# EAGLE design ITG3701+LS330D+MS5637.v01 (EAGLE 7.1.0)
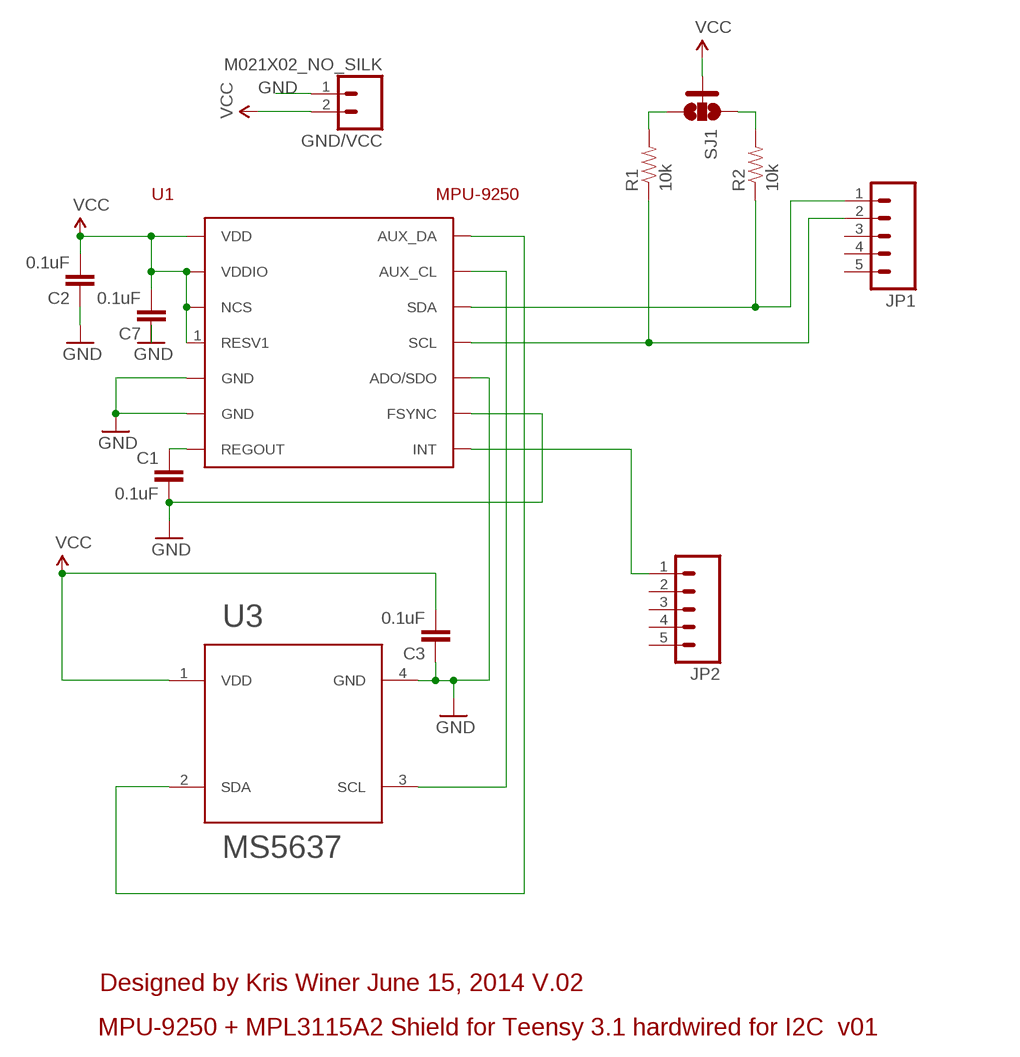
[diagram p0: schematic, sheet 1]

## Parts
C1  0.1uF  4.7UF-6.3V-10%(0603)0603  [0603-CAP]
C2  0.1uF  0.22UF-25V-10%(0603)  [0603-CAP]
C3  0.1uF  0.22UF-25V-10%(0603)  [0603-CAP]
C7  0.1uF  0.22UF-25V-10%(0603)  [0603-CAP]
GND/VCC  M021X02_NO_SILK  [1X02_NO_SILK]
JP1  M05NO_SILK  [1X05_NO_SILK]
JP2  M05NO_SILK  [1X05_NO_SILK]
R1  10k  10K-1%RES-00824  [0603-RES]
R2  10k  10K-1%RES-00824  [0603-RES]
SJ1  SOLDERJUMPER_2WAYS  [SJ_3]
U1  MPU-9250  [MPU-9250]
U3  MS5637  [MS5637QFN-4]

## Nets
GND: C1.2 C2.1 C3.1 C7.1 GND/VCC.1 U1.9(ADO/SDO) U1.11(FSYNC) U1.18(GND) U1.20(GND) U3.4(GND)
N$1: JP1.1 R2.1 U1.24(SDA)
N$2: JP1.2 R1.1 U1.23(SCL)
N$3: C1.1 U1.10(REGOUT)
N$4: JP2.1 U1.12(INT)
N$7: U1.7(AUX_CL) U3.3(SCL)
N$9: R1.2 SJ1.3
N$10: R2.2 SJ1.1
SDO: U1.21(AUX_DA) U3.2(SDA)
VCC: C2.2 C3.2 C7.2 GND/VCC.2 SJ1.2 U1.1(RESV1) U1.8(VDDIO) U1.13(VDD) U1.22(NCS) U3.1(VDD)
Unconnected: JP1.3 JP1.4 JP1.5 JP2.2 JP2.3 JP2.4 JP2.5

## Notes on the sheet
- Designed by Kris Winer June 15, 2014 V.02
- MPU-9250 + MPL3115A2 Shield for Teensy 3.1 hardwired for I2C  v01

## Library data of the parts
C1 = SparkFun-Capacitors:4.7UF-6.3V-10%(0603): CAP-08280; PROD_ID: CAP-08280; VALUE: 4.7uF
C2 C3 C7 = SparkFun-Capacitors:0.22UF-25V-10%(0603): CAP-07822; PROD_ID: CAP-07822; VALUE: 0.22uF
GND/VCC = SparkFun-Connectors:M02: Standard 2-pin 0.1" header. Use with
JP1 JP2 = SparkFun-Connectors:M05: Header 5 Standard 5-pin 0.1" header. Use with straight break away headers (SKU : PRT-00116), right angle break away headers (PRT-00553), swiss pins (PRT-00743), machine pins (PRT-00117), and female headers (PRT-00115). Molex polarized connector foot print use with SKU : PRT-08230 with associated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
R1 R2 = SparkFun-Resistors:10K-1%: 10k-ohm SMT; PROD_ID: RES-00824
SJ1 = SparkFun-Passives:SOLDERJUMPER_2WAY: Solder Jumper 2 way solder jumper
U1 = SparkFun-Sensors:MPU-9250: The MPU-9250 is a 9-axis motion sensor that contains an accelerometer/gyro sensor (MPU-6500) combined with a magnetometer (AK8963).
U3 = SparkFun-DiscreteSemi:MS5637: MS5637 I2C pressure sensor in QFN-4 package by Measurement Specialties

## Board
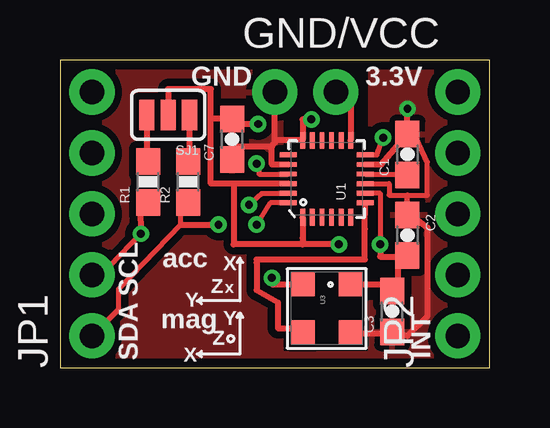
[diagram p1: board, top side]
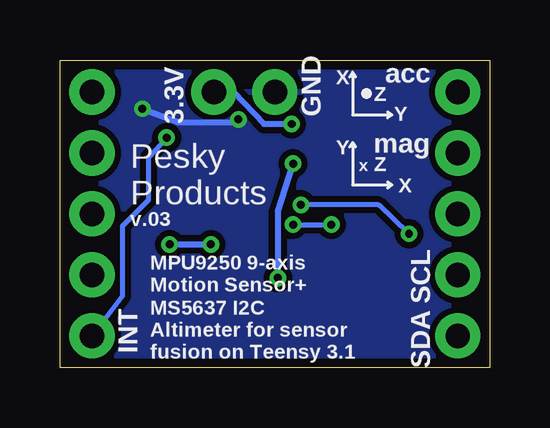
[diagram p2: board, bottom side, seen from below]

Size 17.91 x 12.83 mm. Coordinates in mm from the lower left corner, seen from the top.
Outline: 0,0 17.91,0 17.91,12.83 0,12.83 0,0
Copper layers (1*16): Top 0.0356mm / dielectric 1.5011mm / Bottom 0.0356mm
Design rules "OSHPark *": minimum track width 6mil, minimum drill 13mil, track to track 6mil, track to pad 6mil, pad to pad 6mil, via to via 6mil, smd to smd 6mil, copper to edge 15mil, drill to drill 6mil, minimum pad ring 7mil, minimum via ring 7mil, stop-mask expansion 3mil, vias tented up to drill 20mil, thermal gap 10mil

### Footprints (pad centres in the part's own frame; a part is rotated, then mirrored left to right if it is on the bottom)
0603-CAP = smd 1.1 x 1: 1 -0.85,0; 2 0.85,0
1X02_NO_SILK = drill 1.016 pad 1.88: 1 0,0; 2 2.54,0
1X05_NO_SILK = drill 1.016 pad 1.88: 1 0,0; 2 2.54,0; 3 5.08,0; 4 7.62,0; 5 10.16,0
0603-RES = smd 1.1 x 1: 1 -0.85,0; 2 0.85,0
SJ_3 = smd 0.635 x 1.27: 1 -0.889,0; 2 0,0; 3 0.889,0
MPU-9250 = smd 0.7 x 0.2: 1 -1.6,1; 2 -1.6,0.6; 3 -1.6,0.2; 4 -1.6,-0.2; 5 -1.6,-0.6; 6 -1.6,-1; 13 1.6,-1; 14 1.6,-0.6; 15 1.6,-0.2; 16 1.6,0.2; 17 1.6,0.6; 18 1.6,1 | smd 0.2 x 0.7: 7 -1,-1.6; 8 -0.6,-1.6; 9 -0.2,-1.6; 10 0.2,-1.6; 11 0.6,-1.6; 12 1,-1.6; 19 1,1.6; 20 0.6,1.6; 21 0.2,1.6; 22 -0.2,1.6; 23 -0.6,1.6; 24 -1,1.6
MS5637QFN-4 = smd 1 x 1: 1 -1,1; 2 -1,-1; 3 1,-1; 4 1,1

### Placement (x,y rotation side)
C1  14.48,8.89 90 top
C2  14.48,5.52 270 top
C3  13.84,2.35 90 top
C7  7.18,9.53 90 top
GND/VCC  8.95,11.49 0 top
JP1  1.33,1.33 90 top
JP2  16.57,1.33 90 top
R1  3.67,7.75 90 top
R2  5.35,7.75 90 top
SJ1  4.51,10.54 180 top
U1  11.11,7.87 90 top
U3  11.11,2.48 270 top

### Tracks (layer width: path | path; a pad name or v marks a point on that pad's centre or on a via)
GND  (via drill 0.33)
  Top 0.203: U1.9 13.72,7.67 13.72,7.2 14.48,7.2 | 14.48,7.2 15.3,7.2 15.3,8.57 14.86,9.53 | C2.1 14.48,7.2
  Top 0.254: U1.20 8.83,8.47 8.83,9.21 | v10.48,10.35 10.11,10.35 U1.18 9.02,9.47 8.95,9.4 | U1.11 13.39,8.47 C1.2 | C1.2 v14.48,10.79 | 14.86,9.53 C1.2 | 8.83,9.21 8.95,9.4 | 8.83,9.21 7.24,9.21 C7.1 | 8.95,9.4 GND/VCC.1 | U3.4 12.26,1.44 13.84,1.44 C3.1 13.76,1.33 14.48,1.33 15.3,2.16 15.3,5.84 14.77,6.25 C2.1
  Bottom 0.254: v14.48,10.79 12.95,10.22 10.6,10.22 v10.48,10.35
  pour Bottom (isolate 0.254): 0,12.83 0,0 17.91,0 17.91,12.83
  pour Top (isolate 0.305): 0,0 17.91,0 17.91,12.76 12.95,12.76 12.95,0.57 9.21,0.57 9.21,12.76 0,12.76
N$1  (via drill 0.33)
  Top 0.203: JP1.1 2.44,2.44 2.44,3.28 5.04,5.97 5.04,6.67 R2.1 | v8.19,5.97 8.77,6.87 U1.24
  Top 0.254: 5.04,5.97 v6.6,5.97
  Bottom 0.203: v8.19,5.97 v6.6,5.97
N$2  (via drill 0.33)
  Top 0.203: JP1.2 1.65,4.19 2.1,4.25 v3.37,5.59 | v7.87,6.79 8.4,7.27 U1.23
  Top 0.254: R1.1 3.35,6.66 v3.37,5.59
  Bottom 0.203: v3.37,5.59 4.64,6.79 v7.87,6.79
N$3
  Top 0.203: U1.10 14.7,8.07
  Top 0.254: 14.7,8.07 C1.1
N$4  (via drill 0.33)
  Top 0.203: U1.12 13.21,8.88 v13.46,9.59
  Bottom 0.203: v13.46,9.59 14.22,8.76 14.22,6.99 15.3,5.91 15.3,2.98 JP2.1
N$7
  Top 0.254: U1.7 12.71,5.79 12.71,4.51 8.19,4.51 8.19,4.38 8.19,3.24 9.08,2.73 9.08,1.65 10.1,1.65 U3.3
N$9
  Top 0.254: SJ1.3 3.62,8.95 R1.2
N$10
  Top 0.254: R2.2 5.4,8.79 SJ1.1
SDO  (via drill 0.33)
  Top 0.203: v8.19,8.51 8.3,8.07 U1.21
  Top 0.254: v8.83,3.75 8.83,3.49 U3.2
  Bottom 0.254: v8.19,8.51 8.83,6.48 v8.83,3.75
VCC  (via drill 0.33)
  Top 0.203: v13.34,5.14 13.34,7.27 U1.8
  Top 0.254: GND/VCC.2 12.13,11.49 12.11,11.24 U1.13 | v8.26,10.16 7.39,10.16 C7.2 6.31,10.38 6.29,10.35 | 7.24,7.67 6.29,7.67 6.29,10.35 | 6.29,10.35 6.29,11.62 4.51,11.62 SJ1.2 | 7.24,7.67 7.24,5.14 10.1,5.14 | U1.22 7.24,7.67 | v11.62,5.14 10.1,5.14 | U1.1 10.11,5.41 10.1,5.14 | U3.1 13.44,3.48 C3.2 14.1,3.2 14.1,4.64 | v13.34,5.14 13.34,4.64 14.1,4.64 | 14.1,4.64 14.39,4.64 C2.2 14.1,4.64
  Bottom 0.254: v8.26,10.16 9.4,10.16 10.67,11.49 GND/VCC.2 | v13.34,5.14 v11.62,5.14

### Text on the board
tPlace: GND | 3.3V | acc | X | SCL | Y | Z | x | mag | Y | Z | SDA | X | INT
bPlace: acc | X | Z | mag | Y | GND | 3.3V | Y | Z | x | X | Pesky / Products | v.03 | SCL | MPU9250 9-axis / Motion Sensor+ | SDA | INT | MS5637 I2C / Altimeter for sensor / fusion on Teensy 3.1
